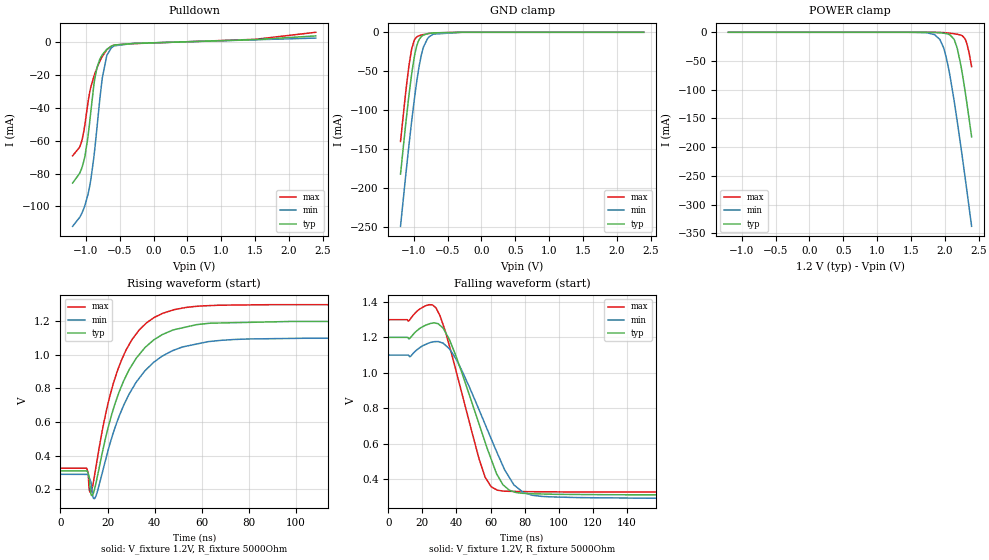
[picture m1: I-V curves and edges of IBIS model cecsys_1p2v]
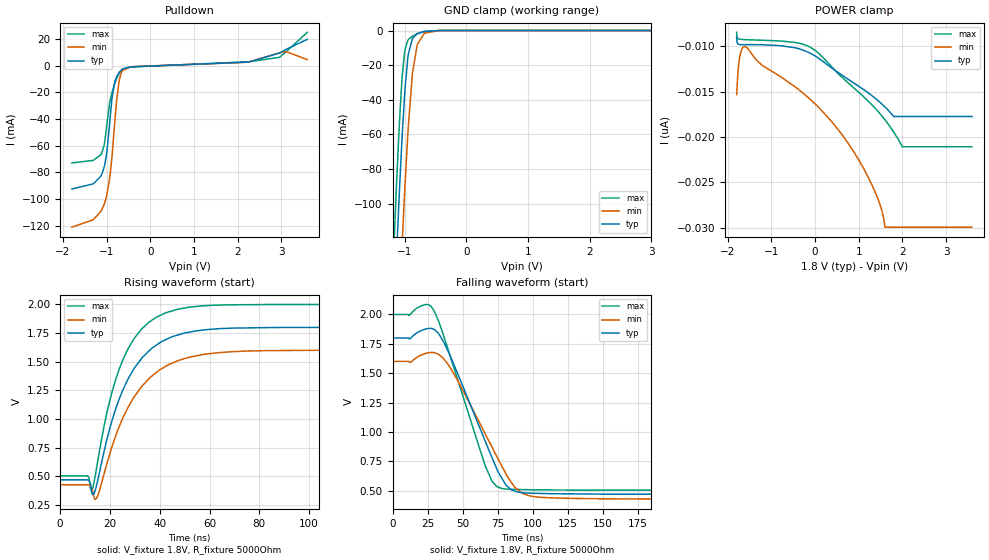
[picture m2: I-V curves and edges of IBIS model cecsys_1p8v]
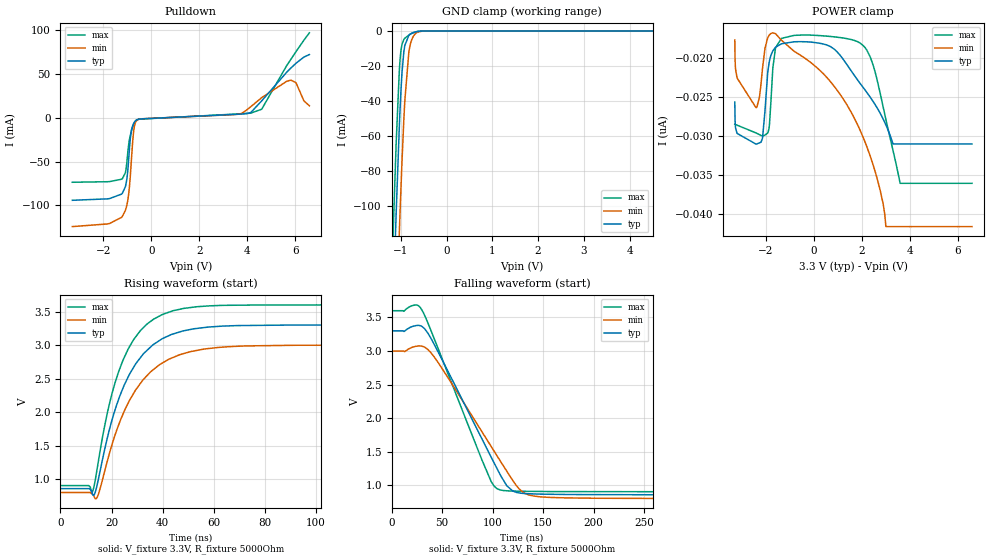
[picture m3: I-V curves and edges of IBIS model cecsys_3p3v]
| Texas Instruments Incorporated
| HDMI Companion Chip with levl shifting buffer 5V load switch
| and ESD protection
| Marketing part#   Voltage Range   Package-type   #pins/pkg drawing
| TDP5S116YFFR   1.1V - 5.5V   YFF   15/WCSP
[IBIS Ver]   4.1
[File name]   tpd5s116.ibs
[File Rev]   1.0
[Date]   10/26/2012
[Source]
| Texas Instruments Incorporated.
| Analog-eLab Design Center, HPA
| 12500 TI Blvd
| Dallas, TX -75243
| e-mail: elab_scm_ibis@list.ti.com
[Notes]   Revision History:
| Rev 1.0: 10/26/2012
| - Initial version of the model
| - Model generated from simulations in TISPICE
| - C_comp although listed in numerical order of value are
|   obtained from varying PVT conditions. For PVT conditions for
|   each specific value refer the buffer description under
|   respective [Model]. IBIS model user is responsible for using
|   appropriate C_comp to simulate for Signal Integrity.
| - POWER and GND clamp Non-monotonic behavior result of buffer design
| - Combined Pullup and Pulldown non-monotonic behavior due to buffer design
[Disclaimer]  This model is designed as an aid for customers of Texas Instruments
 TI and its licensors and suppliers make no warranties, either expressed
 or implied, with respect to this  model, including the warranties of
 merchantability or fitness for a particular purpose.
 The model is provided solely on an "as is" basis. The entire risk as to
 its quality and performance is with the customer.
[Copyright] (C)Copyright 2012 Texas Instruments Incorporated.
   All rights reserved.
[Component]  TPD5S116
[Manufacturer]  Texas Instruments
[Package]   |15 pin WCSP YFF
|   typ   min   max
R_pkg   0   0   0
L_pkg   0   0   0
C_pkg   0   0   0
[Pin]   signal_name   model_name   R_pin   L_pin   C_pin
A1   CECSYS   CECSYS   0.005   0.2nH   0.6pF
A2   VCCA   POWER   0.005   0.2nH   0.6pF
A3   CECCON   ceccon_3v   0.005   0.2nH   0.6pF
B1   SCLSYS   SDASYS   0.005   0.2nH   0.6pF
B2   GND   GND   0.005   0.2nH   0.6pF
B3   SCLCON   sdacon_5v   0.005   0.2nH   0.6pF
C1   SDASYS   SDASYS   0.005   0.2nH   0.6pF
C2   EN   EN   0.005   0.2nH   0.6pF
C3   SDACON   sdacon_5v   0.005   0.2nH   0.6pF
D1   5V_SYS   POWER   0.005   0.2nH   0.6pF
D2   GND   GND   0.005   0.2nH   0.6pF
D3   5V_CON   POWER   0.005   0.2nH   0.6pF
E1   HDPSYS   HDPSYS   0.005   0.2nH   0.6pF
E2   UTICON   hdpcon_5v   0.005   0.2nH   0.6pF
E3   HDPCON   hdpcon_5v   0.005   0.2nH   0.6pF
|   Model Selectors
[Model Selector] CECSYS
cecsys_1p2v  1.2V   cec system output
cecsys_1p5v  1.5V   cec system output
cecsys_1p8v  1.8V   cec system output
cecsys_2p5v  2.5V   cec system output
cecsys_3p3v  3.3V   cec system output
cecsys_5v   5V   cec system output
[Model Selector] SDASYS
sdasys_1p2v  1.2V   cec system output
sdasys_1p5v  1.5V   cec system output
sdasys_1p8v  1.8V   cec system output
sdasys_2p5v  2.5V   cec system output
sdasys_3p3v  3.3V   cec system output
sdasys_5v   5V   cec system output
[Model Selector] HDPSYS
hdpsys_1p2v  1.2V   cec system output
hdpsys_1p5v  1.5V   cec system output
hdpsys_1p8v  1.8V   cec system output
hdpsys_2p5v  2.5V   cec system output
hdpsys_3p3v  3.3V   cec system output
hdpsys_5v   5V   cec system output
[Model Selector] EN
en_1p2v  1.2V   cec system output
en_1p5v  1.5V   cec system output
en_1p8v  1.8V   cec system output
en_2p5v  2.5V   cec system output
en_3p3v  3.3V   cec system output
en_5v   5V   cec system output
| Models and submodels in the file (27): ceccon_3v (I/O_open_drain), cecsys_1p2v (I/O_open_drain), cecsys_1p5v (I/O_open_drain), cecsys_1p8v (I/O_open_drain), cecsys_2p5v (I/O_open_drain), cecsys_3p3v (I/O_open_drain), cecsys_5v (I/O_open_drain), en_1p2v (Input), en_1p5v (Input), en_1p8v (Input), en_2p5v (Input), en_3p3v (Input), en_5v (Input), hdpsys_1p2v (3-state), hdpsys_1p5v (3-state), hdpsys_1p8v (3-state), hdpsys_2p5v (3-state), hdpsys_3p3v (3-state), hdpsys_5v (3-state), hdpcon_5v (Input), sdacon_5v (I/O_open_drain), sdasys_1p2v (I/O_open_drain), sdasys_1p5v (I/O_open_drain), sdasys_1p8v (I/O_open_drain), sdasys_2p5v (I/O_open_drain), sdasys_3p3v (I/O_open_drain), sdasys_5v (I/O_open_drain)
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[Model]   cecsys_1p2v
Model_type   I/O_open_drain
Polarity   Non-Inverting
Enable   Active-Low
Vinl = .0902
Vinh = 0.91
Vmeas = 0.6
Vref = 1.2
Cref = 15pF
Rref = 5000
|   typ   min   max
|   (fast PVT)   (slow PVT)   (nom PVT)
C_comp   1.541p   0.9792p   1.562p
| Where nom  PVT is Nominal Process, 1.2V, 27C
|   Fast PVT is Strong Process,  1.3V, -40C
|   Slow PVT is Weak Process,   1.1V, 125C
[Voltage Range]   1.2   1.1   1.3
[Temperature Range]   27   125   -40
[Pullup Reference]   1.2   1.1   1.3
[Pulldown Reference]   -0   -0   -0
[Power Clamp Reference]   1.2   1.1   1.3
[GND Clamp Reference]   -0   -0   -0
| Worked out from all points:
|   slope of the pulldown table from 0 to 0.18 V, typ, clamps not added: 761 ohm
|   GND clamp passes 1 mA (typ) near -0.74 V on its own axis
|   falling waveform, V_fixture 1.2V, R_fixture 5000Ohm: 20-80 % time 19ns typ, 21.6ns min, 15.9ns max; typ from 1.2 V to 0.308 V
|   rising waveform, V_fixture 1.2V, R_fixture 5000Ohm: 20-80 % time 15.6ns typ, 17.6ns min, 13.7ns max; typ from 0.309 V to 1.2 V
[Pulldown]
|   Voltage   I(typ)   I(min)   I(max)
-1.196V   -85.8mA    -112.2mA   -69.21mA
-1.067V   -77.39mA   -104.8mA   -60.96mA
-1.013V   -69.03mA   -99.3mA    -49.57mA
-969.6mV  -57.65mA   -92.83mA   -36.75mA
-926.4mV  -41.85mA   -83.54mA   -27.13mA
-883.2mV  -26.3mA    -70.4mA    -20.86mA
-836.4mV  -15.39mA   -52.03mA   -15.56mA
-757.2mV  -7.477mA   -21.55mA   -8.494mA
-692.4mV  -4.248mA   -8.171mA   -4.547mA
-609.6mV  -2.016mA   -2.834mA   -1.985mA
1.504V    1.75mA     1.65mA     1.909mA
2.396V    3.994mA    2.674mA    6.208mA
[GND Clamp]
|   Voltage   I(typ)   I(min)   I(max)
-1.196V   -181.9mA   -249mA     -140mA
-1.106V   -107.2mA   -172.8mA   -67mA
-1.067V   -77.35mA   -141.1mA   -40.08mA
-1.027V   -50.76mA   -110.9mA   -19.97mA
-994.8mV  -32.72mA   -87.76mA   -10.59mA
-958.8mV  -18.13mA   -64.41mA   -6.142mA
-890.4mV  -5.71mA    -29.83mA   -3.555mA
-854.4mV  -3.464mA   -18.22mA   -2.835mA
-768mV    -1.332mA   -5.421mA   -1.468mA
-710.4mV  -735.2uA   -2.383mA   -795.9uA
-296.4mV  -134.8nA   -1.36uA    -10.57nA
2.396V    0A         0A         0A
[POWER Clamp]
|   Voltage   I(typ)   I(min)   I(max)
-1.196V   -6.053nA   -9.603nA   -5.733nA
1.5V      -171.4nA   -10.8uA    -16.6nA
1.853V    -362.6uA   -4.393mA   -47.78uA
1.928V    -892uA     -12.58mA   -229uA
1.997V    -1.784mA   -32.39mA   -669.4uA
2.058V    -3.63mA    -63.92mA   -1.336mA
2.144V    -14.06mA   -123.7mA   -2.655mA
2.184V    -27.69mA   -154.7mA   -3.416mA
2.238V    -57.59mA   -199.1mA   -4.98mA
2.296V    -98.83mA   -248.3mA   -10.74mA
2.357V    -148.2mA   -302.1mA   -34.22mA
2.396V    -181.9mA   -337.6mA   -59.75mA
[Ramp]
R_load = 5000
|   typ   min   max
dV/dt_r   0.533284/1.56317e-08   0.487041/1.76118e-08   0.584067/1.36602e-08
dV/dt_f   0.534931/1.89672e-08   0.486885/2.16273e-08   0.585389/1.59107e-08
[Falling Waveform]
V_fixture = 1.2V
V_fixture_min = 1.1V
V_fixture_max = 1.3V
R_fixture = 5000Ohm
C_fixture = 0F
|   Time   V(typ)   V(min)   V(max)
0s        1.2V       1.1V       1.3V
12.67ns   1.195V     1.091V     1.301V
21.22ns   1.266V     1.157V     1.376V
27.94ns   1.28V      1.176V     1.367V
39.43ns   1.102V     1.083V     1.023V
56.8ns    608.4mV    709.5mV    410mV
63.9ns    423.7mV    547.5mV    336.8mV
73.73ns   327.4mV    366.4mV    329.6mV
90.1ns    315.1mV    301.4mV    327.6mV
500ns     308.4mV    288.5mV    324.4mV
[Rising Waveform]
V_fixture = 1.2V
V_fixture_min = 1.1V
V_fixture_max = 1.3V
R_fixture = 5000Ohm
C_fixture = 0F
|   Time   V(typ)   V(min)   V(max)
0s        309mV      288.3mV    324.8mV
11.13ns   308.6mV    288.1mV    324.4mV
12.87ns   175.7mV    244.9mV    180.5mV
13.89ns   171.8mV    149.1mV    233.1mV
15.03ns   231.7mV    157.5mV    327.3mV
21.22ns   617.3mV    479.8mV    767.1mV
27.94ns   876.7mV    731.5mV    1.031V
39.61ns   1.089V     956.1mV    1.222V
53.25ns   1.166V     1.052V     1.283V
500ns     1.198V     1.1V       1.298V
[Model]   cecsys_1p8v
Model_type   I/O_open_drain
Polarity   Non-Inverting
Enable   Active-Low
Vinl = .1312
Vinh = 1.4
Vmeas = 0.9
Vref = 1.8
Cref = 15pF
Rref = 5000
|   typ   min   max
|   (fast PVT)   (slow PVT)   (nom PVT)
C_comp   1.541p   0.9792p   1.562p
| Where nom  PVT is Nominal Process, 1.8V, 27C
|   Fast PVT is Strong Process,  2.0V, -40C
|   Slow PVT is Weak Process,   1.6V, 125C
[Voltage Range]   1.8   1.6   2
[Temperature Range]   27   125   -40
[Pullup Reference]   1.8   1.6   2
[Pulldown Reference]   -0   -0   -0
[Power Clamp Reference]   1.8   1.6   2
[GND Clamp Reference]   -0   -0   -0
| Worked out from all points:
|   slope of the pulldown table from 0 to 0.27 V, typ, clamps not added: 758 ohm
|   GND clamp passes 1 mA (typ) near -0.73 V on its own axis
|   falling waveform, V_fixture 1.8V, R_fixture 5000Ohm: 20-80 % time 27.5ns typ, 30.5ns min, 24ns max; typ from 1.8 V to 0.467 V
|   rising waveform, V_fixture 1.8V, R_fixture 5000Ohm: 20-80 % time 15ns typ, 16.8ns min, 13.2ns max; typ from 0.467 V to 1.8 V
[Pulldown]
|   Voltage   I(typ)   I(min)   I(max)
-1.795V   -92.5mA    -121.1mA   -72.97mA
-1.309V   -88.69mA   -115.6mA   -71.09mA
-1.136V   -83.03mA   -109.5mA   -66.99mA
-1.044V   -74.49mA   -102.8mA   -57.19mA
-995.4mV  -65.08mA   -96.99mA   -44.48mA
-919.8mV  -39.35mA   -81.82mA   -26.14mA
-817.2mV  -12.79mA   -43.98mA   -13.78mA
-714.6mV  -5.3mA     -11.52mA   -5.845mA
-628.2mV  -2.49mA    -3.581mA   -2.504mA
2.255V    2.636mA    2.733mA    2.855mA
2.957V    9.359mA    9.555mA    6.151mA
3.595V    19.64mA    4.455mA    24.91mA
[GND Clamp]
|   Voltage   I(typ)   I(min)   I(max)
-1.795V   -741mA     -803.9mA   -703.2mA
-1.228V   -209.2mA   -276.3mA   -167.3mA
-1.13V    -126.4mA   -192.7mA   -85.32mA
-1.103V   -104.9mA   -170.4mA   -64.8mA
-1.039V   -57.98mA   -119.4mA   -24.85mA
-1.001V   -35.75mA   -91.91mA   -11.85mA
-952.2mV  -16.14mA   -60.45mA   -5.707mA
-876.6mV  -4.671mA   -24.82mA   -3.262mA
-795.6mV  -1.762mA   -7.93mA    -1.861mA
-682.2mV  -530.3uA   -1.536mA   -548.1uA
-444.6mV  -7.005uA   -24.85uA   -2.909uA
3.595V    0A         0A         0A
[POWER Clamp]
|   Voltage   I(typ)   I(min)   I(max)
-1.795V   -8.996nA   -15.31nA   -8.457nA
-1.762V   -9.753nA   -12.78nA   -9.152nA
-1.724V   -9.803nA   -11.2nA    -9.212nA
-1.606V   -9.819nA   -10.02nA   -9.262nA
-1.217V   -9.832nA   -12.07nA   -9.328nA
-217.8mV  -10.52nA   -15.39nA   -9.858nA
532.8mV   -12.9nA    -19.2nA    -13.01nA
1.289V    -15.38nA   -25.12nA   -16.38nA
1.516V    -16.29nA   -27.84nA   -17.58nA
1.602V    -16.68nA   -29.93nA   -18.1nA
2.002V    -17.74nA   -29.93nA   -21.07nA
3.595V    -17.74nA   -29.93nA   -21.07nA
[Ramp]
R_load = 5000
|   typ   min   max
dV/dt_r   0.798364/1.49957e-08   0.705033/1.68238e-08   0.897663/1.31817e-08
dV/dt_f   0.799973/2.74559e-08   0.704838/3.04527e-08   0.898976/2.39986e-08
[Falling Waveform]
V_fixture = 1.8V
V_fixture_min = 1.6V
V_fixture_max = 2V
R_fixture = 5000Ohm
C_fixture = 0F
|   Time   V(typ)   V(min)   V(max)
0s        1.8V       1.6V       2V
23.68ns   1.876V     1.668V     2.085V
29.81ns   1.873V     1.674V     2.028V
39.86ns   1.68V      1.57V      1.693V
66.22ns   917.2mV    980.1mV    708.1mV
70.96ns   779.9mV    869.1mV    578.8mV
77.76ns   609mV      712.7mV    517.8mV
92.28ns   482.6mV    477.7mV    508.2mV
107.6ns   474.7mV    440.9mV    505.5mV
500ns     466.7mV    425.3mV    501.7mV
[Rising Waveform]
V_fixture = 1.8V
V_fixture_min = 1.6V
V_fixture_max = 2V
R_fixture = 5000Ohm
C_fixture = 0F
|   Time   V(typ)   V(min)   V(max)
0s        467.2mV    425mV      502.1mV
11.11ns   467.1mV    424.7mV    502mV
12.77ns   353mV      387.4mV    379.4mV
14.7ns    426.2mV    310.6mV    580.2mV
19.93ns   916.7mV    694.3mV    1.161V
27.44ns   1.355V     1.107V     1.62V
36.86ns   1.618V     1.375V     1.862V
51.99ns   1.758V     1.539V     1.976V
102.5ns   1.799V     1.599V     1.999V
500ns     1.798V     1.6V       1.998V
[Model]   cecsys_3p3v
Model_type   I/O_open_drain
Polarity   Non-Inverting
Enable   Active-Low
Vinl = .246
Vinh = 2.52
Vmeas = 1.65
Vref = 1.65
Cref = 15pF
Rref = 5000
|   typ   min   max
|   (fast PVT)   (slow PVT)   (nom PVT)
C_comp   1.541p   0.9792p   1.562p
| Where nom  PVT is Nominal Process, 3.3V, 27C
|   Fast PVT is Strong Process,  3.6V, -40C
|   Slow PVT is Weak Process,   3.0V, 125C
[Voltage Range]   3.3   3   3.6
[Temperature Range]   27   125   -40
[Pullup Reference]   3.3   3   3.6
[Pulldown Reference]   -0   -0   -0
[Power Clamp Reference]   3.3   3   3.6
[GND Clamp Reference]   -0   -0   -0
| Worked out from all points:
|   slope of the pulldown table from 0 to 0.495 V, typ, clamps not added: 757 ohm
|   GND clamp passes 1 mA (typ) near -0.74 V on its own axis
|   falling waveform, V_fixture 3.3V, R_fixture 5000Ohm: 20-80 % time 49.1ns typ, 55.1ns min, 42.3ns max; typ from 3.3 V to 0.86 V
|   rising waveform, V_fixture 3.3V, R_fixture 5000Ohm: 20-80 % time 14.5ns typ, 16.1ns min, 12.7ns max; typ from 0.86 V to 3.3 V
[Pulldown]
|   Voltage   I(typ)   I(min)   I(max)
-3.29V    -94.27mA   -124.3mA   -73.65mA
-1.201V   -86.01mA   -112.4mA   -69.38mA
-1.063V   -76.97mA   -104.5mA   -60.48mA
-973.5mV  -59.01mA   -93.59mA   -38.16mA
-825mV    -14.05mA   -47.37mA   -14.85mA
-706.2mV  -5.214mA   -10.36mA   -5.715mA
-547.8mV  -1.711mA   -1.957mA   -1.807mA
3.62V     4.14mA     4.094mA    4.502mA
4.145V    5.998mA    12.69mA    5.368mA
4.6V      19.32mA    23.06mA    9.825mA
5.828V    57.17mA    43mA       67.26mA
6.59V     72.39mA    13.8mA     97.2mA
[GND Clamp]
|   Voltage   I(typ)   I(min)   I(max)
-3.29V    -2.207A    -2.262A    -2.175A
-1.201V   -186.1mA   -253.2mA   -144.2mA
-1.152V   -143.9mA   -210.6mA   -102.4mA
-1.102V   -103.9mA   -169.4mA   -63.93mA
-1.033V   -54.32mA   -115.1mA   -22.31mA
-1.003V   -37mA      -93.59mA   -12.41mA
-973.5mV  -23.33mA   -73.6mA    -7.442mA
-914.1mV  -8.309mA   -40.07mA   -4.147mA
-825mV    -2.426mA   -11.99mA   -2.324mA
-755.7mV  -1.178mA   -4.574mA   -1.307mA
-448.8mV  -7.721uA   -26.85uA   -3.288uA
6.59V     0A         0A         0A
[POWER Clamp]
|   Voltage   I(typ)   I(min)   I(max)
-3.29V    -25.61nA   -17.69nA   -28.46nA
-3.191V   -29.63nA   -22.56nA   -28.58nA
-2.409V   -31nA      -26.33nA   -29.57nA
-2.132V   -30.13nA   -21.2nA    -29.98nA
-1.865V   -20.66nA   -17.11nA   -28.98nA
-1.587V   -18.61nA   -16.9nA    -18.66nA
541.2mV   -18.32nA   -22.46nA   -17.19nA
1.521V    -21.46nA   -26.71nA   -17.6nA
2.373V    -25.09nA   -32.71nA   -20nA
3.006V    -28.55nA   -41.55nA   -27.84nA
3.6V      -30.98nA   -41.55nA   -36.01nA
6.59V     -30.98nA   -41.55nA   -36.01nA
[Ramp]
R_load = 5000
|   typ   min   max
dV/dt_r   1.46271/1.45064e-08   1.31854/1.61356e-08   1.6155/1.26936e-08
dV/dt_f   1.46424/4.91054e-08   1.3183/5.51153e-08   1.61662/4.23293e-08
[Falling Waveform]
V_fixture = 3.3V
V_fixture_min = 3V
V_fixture_max = 3.6V
R_fixture = 5000Ohm
C_fixture = 0F
|   Time   V(typ)   V(min)   V(max)
0s        3.3V       3V         3.6V
22.77ns   3.374V     3.066V     3.685V
28.68ns   3.375V     3.075V     3.642V
42.32ns   3.093V     2.908V     3.176V
98.58ns   1.419V     1.579V     1.057V
107.5ns   1.16V      1.365V     932.6mV
119.7ns   918.4mV    1.079V     917.1mV
129.2ns   883.1mV    908.3mV    913.3mV
147.3ns   870.8mV    830.3mV    910.6mV
500ns     859.6mV    802.8mV    905.6mV
[Rising Waveform]
V_fixture = 3.3V
V_fixture_min = 3V
V_fixture_max = 3.6V
R_fixture = 5000Ohm
C_fixture = 0F
|   Time   V(typ)   V(min)   V(max)
0s        860mV      802.5mV    906mV
11.11ns   859.8mV    802.4mV    905.9mV
12.51ns   787mV      775.4mV    810.9mV
14.72ns   976.8mV    761.6mV    1.238V
19.35ns   1.766V     1.409V     2.152V
26.59ns   2.532V     2.142V     2.948V
36.22ns   3.005V     2.63V      3.38V
48.25ns   3.214V     2.874V     3.548V
92.76ns   3.299V     2.999V     3.6V
500ns     3.298V     3V         3.599V
